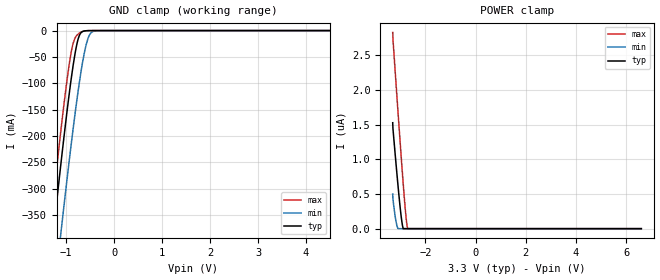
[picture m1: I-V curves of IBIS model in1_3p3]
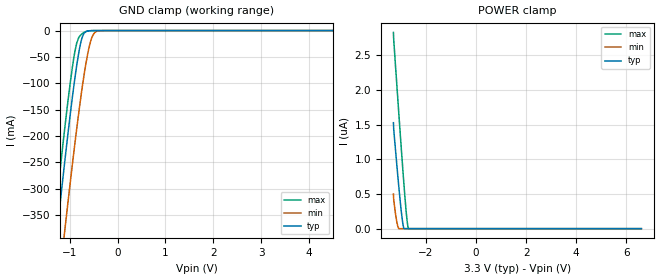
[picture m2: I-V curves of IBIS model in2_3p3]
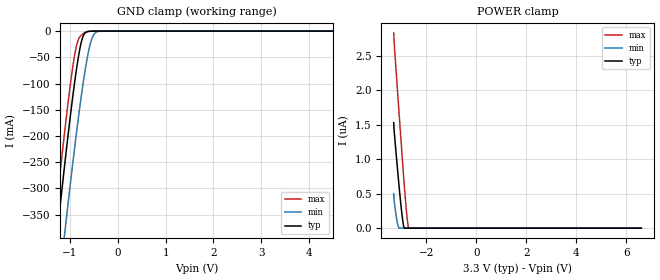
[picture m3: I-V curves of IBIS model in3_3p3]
|Texas Instruments Incorporated
|TLIN2441X Automotive Local Interconnect Network(LIN) Transceiver with
|Integrated Voltage Regulator and Watchdog
[IBIS Ver]   4.1
[File name]   tlin2441x.ibs
[Date]   12/20/2018
[File Rev]   1.0
[Source]
| Texas Instruments Incorporated.
| Analog-eLab Design Center, HPA
| 12500 TI Blvd
| Dallas, TX -75243
[Notes]   Revision History:
| Rev 1.0: 12/20/2018
| - Initial version of the model
| - Model generated from simulations in SPECTRE
| - Model names with a trailing _3p3 contain the model for 3.3V operation.
|   Model names with a trailing _5p0 contain the model for 5.0V operation.
|   Model names with a trailing _14p0 contain the model for 14.0V operation.
|   Model names with a trailing _26p0 contain the model for 26.0V operation.
|   Model names with a trailing _34p0 contain the model for 34.0V operation.
| - C_comp although listed in numerical order of value are
|   obtained from varying PVT conditions. For PVT conditions for
|   each specific value refer the buffer description under
|   respective [Model]. IBIS model user is responsible for using
|   appropriate C_comp to simulate for Signal Integrity.
| - TLIN24415 use VCC = 5p0V/3p3V
| - TLIN24413 use VCC = 3p3V
[Disclaimer]
| This model is designed as an aid for customers of Texas Instruments.
| TI and its licensors and suppliers make no warranties, either expressed
| or implied, with respect to this  model, including the warranties of
| merchantability or fitness for a particular purpose. The model is
| provided solely on an "as is" basis. The entire risk as to its quality
| and performance is with the customer.
| This model is subject to change without notice. Texas Instruments
| Incorporated is not responsible for updating this model.
[Copyright]
(C) Copyright 2018 Texas Instruments Incorporated.All rights reserved.
|  Component TLIN24415DMT 14-Pin VSON -DMT package
|  Part # TLIN24415DMT
[Component]   TLIN24415DMT
[Manufacturer]   TI
[Package]   |14 VSON -DMT package
|   typ   min   max
R_pkg   0.05   0.04   0.06
L_pkg   1.0nH   0.8nH   1.2nH
C_pkg   0.2pF   0.16pF   0.24pF
[Pin] signal_name  model_name   R_pin   L_pin   C_pin
1   VSUP   POWER   NA   NA   NA
2   LIMP   OOS   NA   NA   NA
3   EN/nINT   IOOD1   NA   NA   NA
4   GND   GND   NA   NA   NA
5   LIN   IOOD2   NA   NA   NA
6   WDT/CLK   IN4   NA   NA   NA
7   nWDR/SDO   OUT_OD   NA   NA   NA
8   WDI/SDI   IN1   NA   NA   NA
9   PIN/nCS   IN2   NA   NA   NA
10   RXD   OOD1   NA   NA   NA
11   TXD   IN3   NA   NA   NA
12   nRST/nWDR   OOD2   NA   NA   NA
13   WAKE   IN5   NA   NA   NA
14   VCC   POWER   NA   NA   NA
|  Component TLIN24413DMT 14-Pin VSON -DMT package
|  Part # TLIN24413DMT
[Component]   TLIN24413DMT
[Manufacturer]   TI
[Package]   |14 VSON -DMT package
|   typ   min   max
R_pkg   0.05   0.04   0.06
L_pkg   1.0nH   0.8nH   1.2nH
C_pkg   0.2pF   0.16pF   0.24pF
[Pin] signal_name  model_name   R_pin   L_pin   C_pin
1   VSUP   POWER   NA   NA   NA
2   LIMP   OOS   NA   NA   NA
3   EN/nINT   IOOD1   NA   NA   NA
4   GND   GND   NA   NA   NA
5   LIN   IOOD2   NA   NA   NA
6   WDT/CLK   IN4   NA   NA   NA
7   nWDR/SDO   OUT_OD   NA   NA   NA
8   WDI/SDI   IN1   NA   NA   NA
9   PIN/nCS   IN2   NA   NA   NA
10   RXD   OOD1   NA   NA   NA
11   TXD   IN3   NA   NA   NA
12   nRST/nWDR   OOD2   NA   NA   NA
13   WAKE   IN5   NA   NA   NA
14   VCC   POWER   NA   NA   NA
|   Model Selectors
[Model Selector] IN1
in1_3p3   3.3V   digital Input
in1_5p0   5.0V   digital Input
[Model Selector] IN2
in2_3p3   3.3V   digital Input
in2_5p0   5.0V   digital Input
[Model Selector] IN3
in3_3p3   3.3V   digital Input
in3_5p0   5.0V   digital Input
[Model Selector] IN4
in4_3p3   3.3V   digital Input
in4_5p0   5.0V   digital Input
[Model Selector] IN5
in5_6p0   6.0V   digital Input
in5_14p0   14.0V   digital Input
in5_26p0   26.0V   digital Input
in5_34p0   34.0V   digital Input
[Model Selector] IOOD1
iood1_3p3   3.3V   digital Input
iood1_5p0   5.0V   digital Input
[Model Selector] IOOD2
iood2_6p0   6.0V   digital Input
iood2_14p0   14.0V   digital Input
iood2_26p0   26.0V   digital Input
iood2_34p0   34.0V   digital Input
[Model Selector] OOD1
ood1_3p3   3.3V   digital Input
ood1_5p0   5.0V   digital Input
[Model Selector] OOD2
ood2_3p3   3.3V   digital Input
ood2_5p0   5.0V   digital Input
[Model Selector] OUT_OD
ood3_3p3   3.3V   digital Input Open Drain Mode
ood3_5p0   5.0V   digital Input Open Drain Mode
out_3p3   3.3V   digital Input Output Mode
out_5p0   5.0V   digital Input Output Mode
[Model Selector] OOS
oos_6p0   6.0V   digital Input
oos_14p0   14.0V   digital Input
oos_26p0   26.0V   digital Input
oos_34p0   34.0V   digital Input
| Models and submodels in the file (30): in1_3p3 (Input), in1_5p0 (Input), in2_3p3 (Input), in2_5p0 (Input), in3_3p3 (Input), in3_5p0 (Input), in4_3p3 (Input), in4_5p0 (Input), in5_6p0 (Input), in5_14p0 (Input), in5_26p0 (Input), in5_34p0 (Input), iood1_3p3 (I/O_open_drain), iood1_5p0 (I/O_open_drain), iood2_6p0 (I/O_open_drain), iood2_14p0 (I/O_open_drain), iood2_26p0 (I/O_open_drain), iood2_34p0 (I/O_open_drain), oos_6p0 (Open_source), oos_14p0 (Open_source), oos_26p0 (Open_source), oos_34p0 (Open_source), ood1_3p3 (Open_drain), ood1_5p0 (Open_drain), ood2_3p3 (Open_drain), ood2_5p0 (Open_drain), ood3_3p3 (Open_drain), ood3_5p0 (Open_drain), out_3p3 (3-state), out_5p0 (3-state)
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|   in1_3p3 Model
[Model]   in1_3p3
Model_type   Input
Vinl = 0.8
Vinh = 2.19
|   typ   min   max
C_comp   4.504pF   4.362pF   4.525pF
|  Where Nom  PVT is Nominal Process, 3.3V,   27C
|   Fast PVT is Strong Process,  3.6,   -40C
|   Slow PVT is Weak Process,   3.0V,   150C
[Voltage Range]   3.3   3   3.6
|Junction Temperature
[Temperature Range]   27   150   -40
[Power Clamp Reference]   3.3   3   3.6
[GND Clamp Reference]   0   0   0
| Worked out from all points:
|   GND clamp passes 1 mA (typ) near -0.63 V on its own axis
[GND Clamp]
|   Voltage   I(typ)   I(min)   I(max)
-3.3V     -2.208A    -2.294A    -2.167A
-1.33V    -437mA     -566.9mA   -373.8mA
-1.231V   -353.1mA   -484mA     -289.3mA
-1.102V   -247.3mA   -378.4mA   -183.9mA
-983.4mV  -154.8mA   -283.9mA   -95.2mA
-884.4mV  -85.28mA   -208.5mA   -36.2mA
-775.5mV  -25.56mA   -131.6mA   -8.893mA
-676.5mV  -2.938mA   -70.74mA   -2.425mA
-597.3mV  -421uA     -32.6mA    -493.6uA
-537.9mV  -105uA     -13.42mA   -119.2uA
-399.3mV  -15.24uA   -536.4uA   -16.65uA
6.6V      0A         0A         0A
[POWER Clamp]
|   Voltage   I(typ)   I(min)   I(max)
-3.3V     1.529uA    500.7nA    2.833uA
-3.29V    1.444uA    425.7nA    2.739uA
-3.231V   1.194uA    252.3nA    2.424uA
-3.132V   789.5nA    44.01nA    1.906uA
-3.092V   633.5nA    2.114nA    1.701uA
-3.003V   305.8nA    0A         1.244uA
-2.944V   122.8nA    0A         947.3nA
-2.884V   2.864nA    0A         659.4nA
-2.795V   0A         0A         263.5nA
-2.746V   0A         0A         89.32nA
-2.706V   0A         0A         3.64nA
6.6V      0A         0A         0A
|   in2_3p3 Model
[Model]   in2_3p3
Model_type   Input
Vinl = 0.8
Vinh = 2.19
|   typ   min   max
C_comp   4.504pF   4.302pF   4.525pF
|  Where Nom  PVT is Nominal Process, 3.3V,   27C
|   Fast PVT is Strong Process,  3.6,   -40C
|   Slow PVT is Weak Process,   3.0V,   150C
[Voltage Range]   3.3   3   3.6
|Junction Temperature
[Temperature Range]   27   150   -40
[Power Clamp Reference]   3.3   3   3.6
[GND Clamp Reference]   0   0   0
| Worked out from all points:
|   GND clamp passes 1 mA (typ) near -0.63 V on its own axis
[GND Clamp]
|   Voltage   I(typ)   I(min)   I(max)
-3.3V     -2.208A    -2.294A    -2.167A
-1.33V    -437mA     -566.9mA   -373.8mA
-1.231V   -353.1mA   -484mA     -289.3mA
-1.102V   -247.3mA   -378.4mA   -183.9mA
-983.4mV  -154.8mA   -283.9mA   -95.2mA
-884.4mV  -85.28mA   -208.5mA   -36.2mA
-775.5mV  -25.56mA   -131.6mA   -8.893mA
-676.5mV  -2.938mA   -70.74mA   -2.425mA
-597.3mV  -421uA     -32.6mA    -493.6uA
-537.9mV  -105uA     -13.42mA   -119.2uA
-399.3mV  -15.24uA   -536.4uA   -16.65uA
6.6V      0A         0A         0A
[POWER Clamp]
|   Voltage   I(typ)   I(min)   I(max)
-3.3V     1.529uA    500.7nA    2.833uA
-3.29V    1.444uA    425.7nA    2.739uA
-3.231V   1.194uA    252.3nA    2.424uA
-3.132V   789.5nA    44.01nA    1.906uA
-3.092V   633.5nA    2.114nA    1.701uA
-3.003V   305.8nA    0A         1.244uA
-2.944V   122.8nA    0A         947.3nA
-2.884V   2.864nA    0A         659.4nA
-2.795V   0A         0A         263.5nA
-2.746V   0A         0A         89.32nA
-2.706V   0A         0A         3.64nA
6.6V      0A         0A         0A
|   in3_3p3 Model
[Model]   in3_3p3
Model_type   Input
Vinl = 0.8
Vinh = 2
|   typ   min   max
C_comp   4.504pF   4.302pF   4.525pF
|  Where Nom  PVT is Nominal Process, 3.3V,   27C
|   Fast PVT is Strong Process,  3.6,   -40C
|   Slow PVT is Weak Process,   3.0V,   150C
[Voltage Range]   3.3   3   3.6
|Junction Temperature
[Temperature Range]   27   150   -40
[Power Clamp Reference]   3.3   3   3.6
[GND Clamp Reference]   0   0   0
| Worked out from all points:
|   GND clamp passes 1 mA (typ) near -0.63 V on its own axis
[GND Clamp]
|   Voltage   I(typ)   I(min)   I(max)
-3.3V     -2.208A    -2.294A    -2.167A
-1.33V    -437mA     -566.9mA   -373.8mA
-1.231V   -353.1mA   -484mA     -289.3mA
-1.102V   -247.3mA   -378.4mA   -183.9mA
-983.4mV  -154.8mA   -283.9mA   -95.2mA
-884.4mV  -85.28mA   -208.5mA   -36.2mA
-775.5mV  -25.56mA   -131.6mA   -8.893mA
-676.5mV  -2.938mA   -70.74mA   -2.425mA
-597.3mV  -421uA     -32.6mA    -493.6uA
-537.9mV  -105uA     -13.42mA   -119.2uA
-399.3mV  -15.24uA   -536.4uA   -16.65uA
6.6V      0A         0A         0A
[POWER Clamp]
|   Voltage   I(typ)   I(min)   I(max)
-3.3V     1.529uA    500.7nA    2.833uA
-3.29V    1.444uA    425.7nA    2.739uA
-3.231V   1.194uA    252.3nA    2.424uA
-3.132V   789.5nA    44.01nA    1.906uA
-3.092V   633.5nA    2.114nA    1.701uA
-3.003V   305.8nA    0A         1.244uA
-2.944V   122.8nA    0A         947.3nA
-2.884V   2.864nA    0A         659.4nA
-2.795V   0A         0A         263.5nA
-2.746V   0A         0A         89.32nA
-2.706V   0A         0A         3.64nA
6.6V      0A         0A         0A
